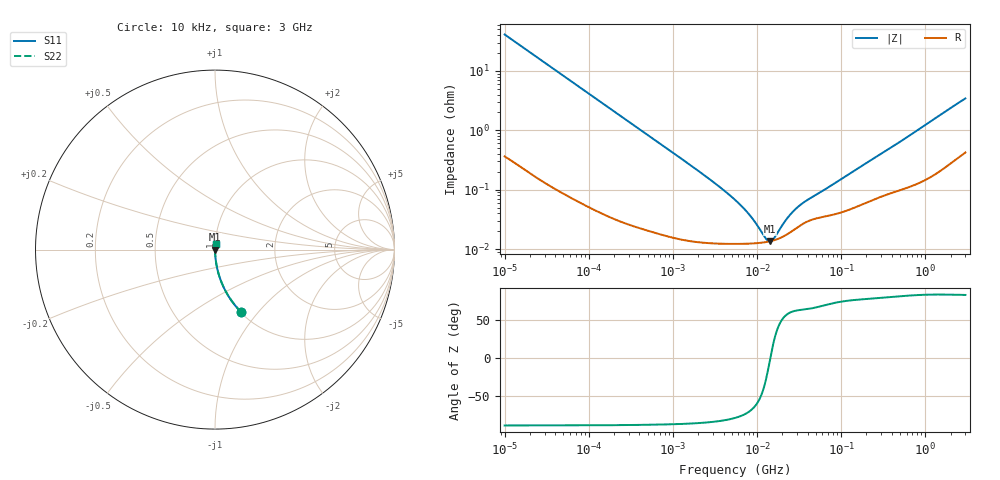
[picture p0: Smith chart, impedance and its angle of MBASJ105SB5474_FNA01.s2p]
! MBASJ105SB5474_FNA01  S-PARAMETER MODEL  ( Standard Model )
! Model Generated by TAIYO YUDEN Corporation (http://www.ty-top.com)
! Version 1.0
! TAIYO YUDEN Control No. 220601
! Copyright(c) 2013 TAIYO YUDEN CO.,LTD. All Rights Reserved.
! Product Description (link to TY-COMPAS)
! https://ds.yuden.co.jp/TYCOMPAS/or/detail?pn=MBASJ105SB5474KFNA01&u=M
! Products Name : Multilayer Ceramic Capacitors
! Characteristics :
!  Capacitance : 0.47 [uF] , Rated Voltage : 6.3 [V] , TCC : X5R
!  Case Size : 1.0 x 0.5 / 0.039 x 0.02 [mm/inch] , Thickness : 0.5 / 0.02 [mm/inch]
!  (Conditions: Temperature = 25 [degC] , DC Bias Voltage = 0 [V])
! External Node Assignments :
!  1  o---| |---o  2
! GND o---------o GND
! Frequency Range : 10kHz  -  3GHz  [ 401 STEP ]
# MHZ S RI R 50
! Freq[MHz].  S11 Real  S11 Imag  S21 Real  S21 Imag  S12 Real  S12 Imag  S22 Real  S22 Imag
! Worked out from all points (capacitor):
!   401 points, 10 kHz to 3 GHz, reference 50 ohm
!   read as one part in series: C = 388 nF near 10.65 kHz
!   lowest |Z| = 13.6 mohm at 14.1 MHz (marker M1)
!   series resonance near 14.44 MHz, so ESL is about 310 pH
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0.01  0.1459 -0.3486  0.8541 0.3486  0.8541 0.3486  0.1459 -0.3486
0.016047  0.0635 -0.2393  0.9365 0.2393  0.9365 0.2393  0.0635 -0.2393
0.027426  0.0234 -0.1465  0.9766 0.1465  0.9766 0.1465  0.0234 -0.1465
0.045421  0.00911 -0.0901  0.9909 0.0901  0.9909 0.0901  0.00911 -0.0901
0.082683  0.00309 -0.05  0.9969 0.05  0.9969 0.05  0.00309 -0.05
0.199902  0.000755 -0.0208  0.9992 0.0208  0.9992 0.0208  0.000755 -0.0208
0.683653  0.000217 -0.00614  0.9998 0.00614  0.9998 0.00614  0.000217 -0.00614
2.652321  0.000128 -0.00154  0.9999 0.00154  0.9999 0.00154  0.000128 -0.00154
5.477226  0.000123 -0.000664  0.9999 0.000664  0.9999 0.000664  0.000123 -0.000664
7.996027  0.000124 -0.00037  0.9999 0.00037  0.9999 0.00037  0.000124 -0.00037
9.6612  0.000126 -0.000244  0.9999 0.000244  0.9999 0.000244  0.000126 -0.000244
12.43293  0.000131 -8.9e-05  0.9999 8.9e-05  0.9999 8.9e-05  0.000131 -8.9e-05
13.24217  0.000133 -5.13e-05  0.9999 5.13e-05  0.9999 5.13e-05  0.000133 -5.13e-05
14.10408  0.000135 -1.38e-05  0.9999 1.38e-05  0.9999 1.38e-05  0.000135 -1.38e-05
15.02209  0.000138 2.37e-05  0.9999 -2.37e-05  0.9999 -2.37e-05  0.000138 2.37e-05
15.99985  0.000141 6.12e-05  0.9999 -6.12e-05  0.9999 -6.12e-05  0.000141 6.12e-05
21.93027  0.000172 0.000253  0.9998 -0.000253  0.9998 -0.000253  0.000172 0.000253
27.34599  0.000211 0.000388  0.9998 -0.000388  0.9998 -0.000388  0.000211 0.000388
34.09912  0.00026 0.000517  0.9997 -0.000517  0.9997 -0.000517  0.00026 0.000517
45.28751  0.000314 0.000684  0.9997 -0.000684  0.9997 -0.000684  0.000314 0.000684
374.4521  0.000877 0.00483  0.9991 -0.00483  0.9991 -0.00483  0.000877 0.00483
3000  0.00536 0.0338  0.9946 -0.0338  0.9946 -0.0338  0.00536 0.0338
